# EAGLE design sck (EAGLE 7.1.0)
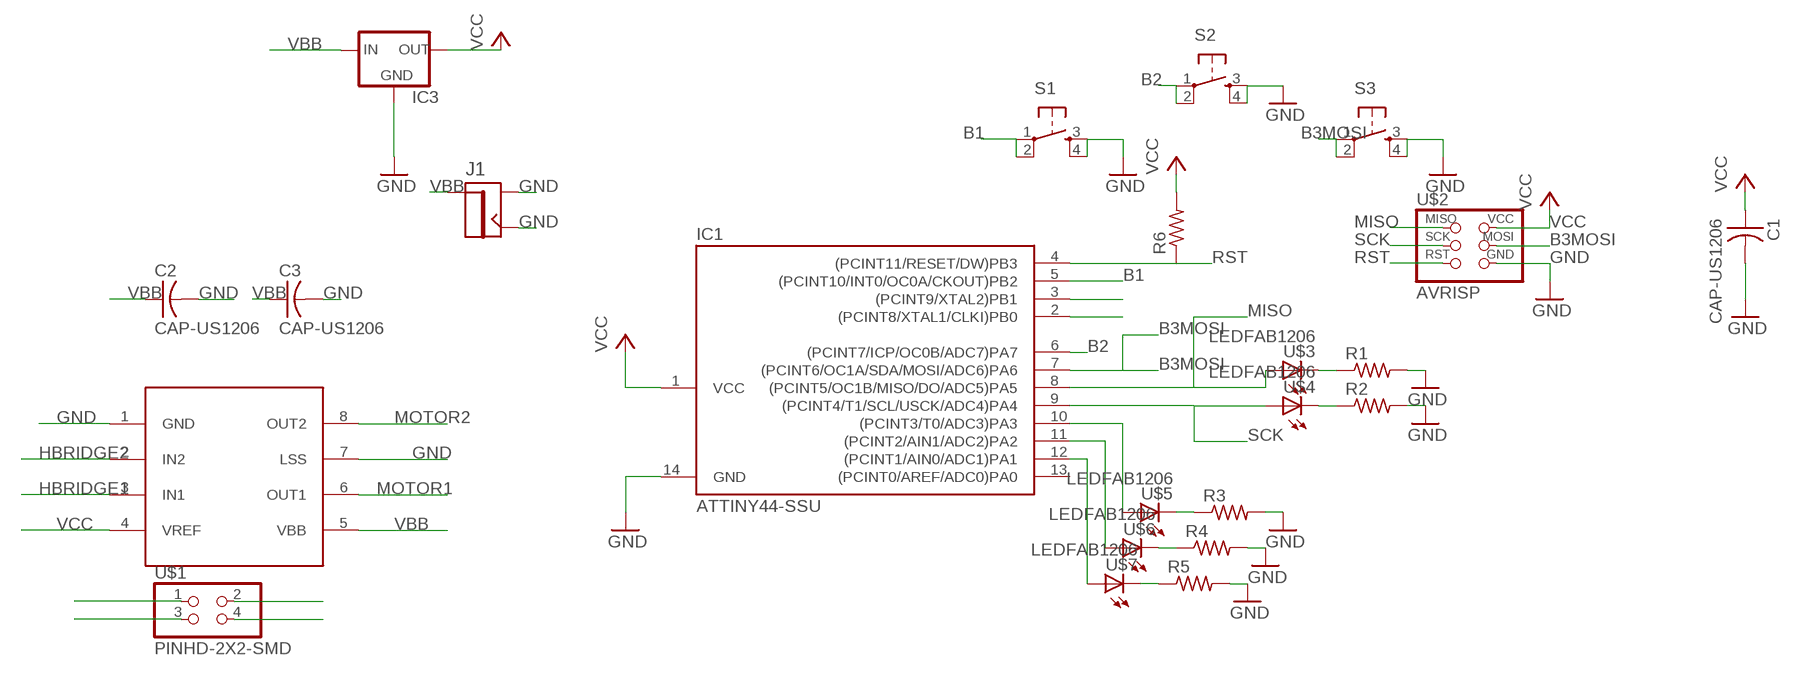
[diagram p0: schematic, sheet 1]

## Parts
C1  CAP-US1206  [C1206]
C2  CAP-US1206  [C1206]
C3  CAP-US1206  [C1206]
IC1  ATTINY44-SSU  [SOIC14]
IC3  78XXS  [78XXS]
J1  JACK2.1MM  [JACK_2.1MM]
R1  RES-US1206  [R1206]
R2  RES-US1206  [R1206]
R3  RES-US1206  [R1206]
R4  RES-US1206  [R1206]
R5  RES-US1206  [R1206]
R6  RES-US1206  [R1206]
S1  6MM_SWITCH6MM_SWITCH  [6MM_SWITCH]
S2  6MM_SWITCH6MM_SWITCH  [6MM_SWITCH]
S3  6MM_SWITCH6MM_SWITCH  [6MM_SWITCH]
U$1  PINHD-2X2-SMD  [2X02SMD]
U$2  AVRISP  [2X03]
U$3  LEDFAB1206  [LED1206FAB]
U$4  LEDFAB1206  [LED1206FAB]
U$5  LEDFAB1206  [LED1206FAB]
U$6  LEDFAB1206  [LED1206FAB]
U$7  LEDFAB1206  [LED1206FAB]
U$8  A4953-H-BRIDGE-MOTOR-DRIVER  [SOIC8]

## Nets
B1: IC1.5((PCINT10/INT0/OC0A/CKOUT)PB2) S1.1(P) S1.2(P1)
B2: IC1.6((PCINT7/ICP/OC0B/ADC7)PA7) S2.1(P) S2.2(P1)
B3MOSI: IC1.7((PCINT6/OC1A/SDA/MOSI/ADC6)PA6) S3.1(P) S3.2(P1) U$2.4(MOSI)
GND: C1.2 C2.2 C3.2 IC1.14(GND) IC3.GND J1.CONTACT J1.SHUNT R1.2 R2.2 R3.2 R4.2 R5.2 S1.3(S) S1.4(S1) S2.3(S) S2.4(S1) S3.3(S) S3.4(S1) U$2.6(GND) U$8.1(GND) U$8.7(LSS)
HBRIDGE1: IC1.2((PCINT8/XTAL1/CLKI)PB0) U$8.3(IN1)
HBRIDGE2: IC1.3((PCINT9/XTAL2)PB1) U$8.2(IN2)
MISO: IC1.8((PCINT5/OC1B/MISO/DO/ADC5)PA5) U$2.1(MISO) U$3.1(A)
MOTOR1: U$1.1 U$1.2 U$8.6(OUT1)
MOTOR2: U$1.3 U$1.4 U$8.8(OUT2)
N$1: R1.1 U$3.2(C)
N$2: R2.1 U$4.2(C)
N$3: R3.1 U$5.2(C)
N$4: R4.1 U$6.2(C)
N$5: R5.1 U$7.2(C)
N$6: IC1.12((PCINT1/AIN0/ADC1)PA1) U$7.1(A)
N$7: IC1.11((PCINT2/AIN1/ADC2)PA2) U$6.1(A)
N$8: IC1.10((PCINT3/T0/ADC3)PA3) U$5.1(A)
RST: IC1.4((PCINT11/RESET/DW)PB3) R6.1 U$2.5(RST)
SCK: IC1.9((PCINT4/T1/SCL/USCK/ADC4)PA4) U$2.3(SCK) U$4.1(A)
VBB: C2.1 C3.1 IC3.IN J1.PIN U$8.5(VBB)
VCC: C1.1 IC1.1(VCC) IC3.OUT R6.2 U$2.2(VCC) U$8.4(VREF)
Unconnected: IC1.13((PCINT0/AREF/ADC0)PA0)

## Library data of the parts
C1-C3 = fab:CAP-US
IC1 = fab:ATTINY44
IC3 = v-reg:78XXS: VOLTAGE REGULATOR
J1 = fab:JACK
R1-R6 = fab:RES-US: Resistor (US Symbol)
S1-S3 = fab:6MM_SWITCH: OMRON SWITCH
U$1 = fab:PINHD-2X2-SMD
U$2 = fab:AVRISP
U$3-U$7 = fab:LED: LED
U$8 = fab:A4953-H-BRIDGE-MOTOR-DRIVER

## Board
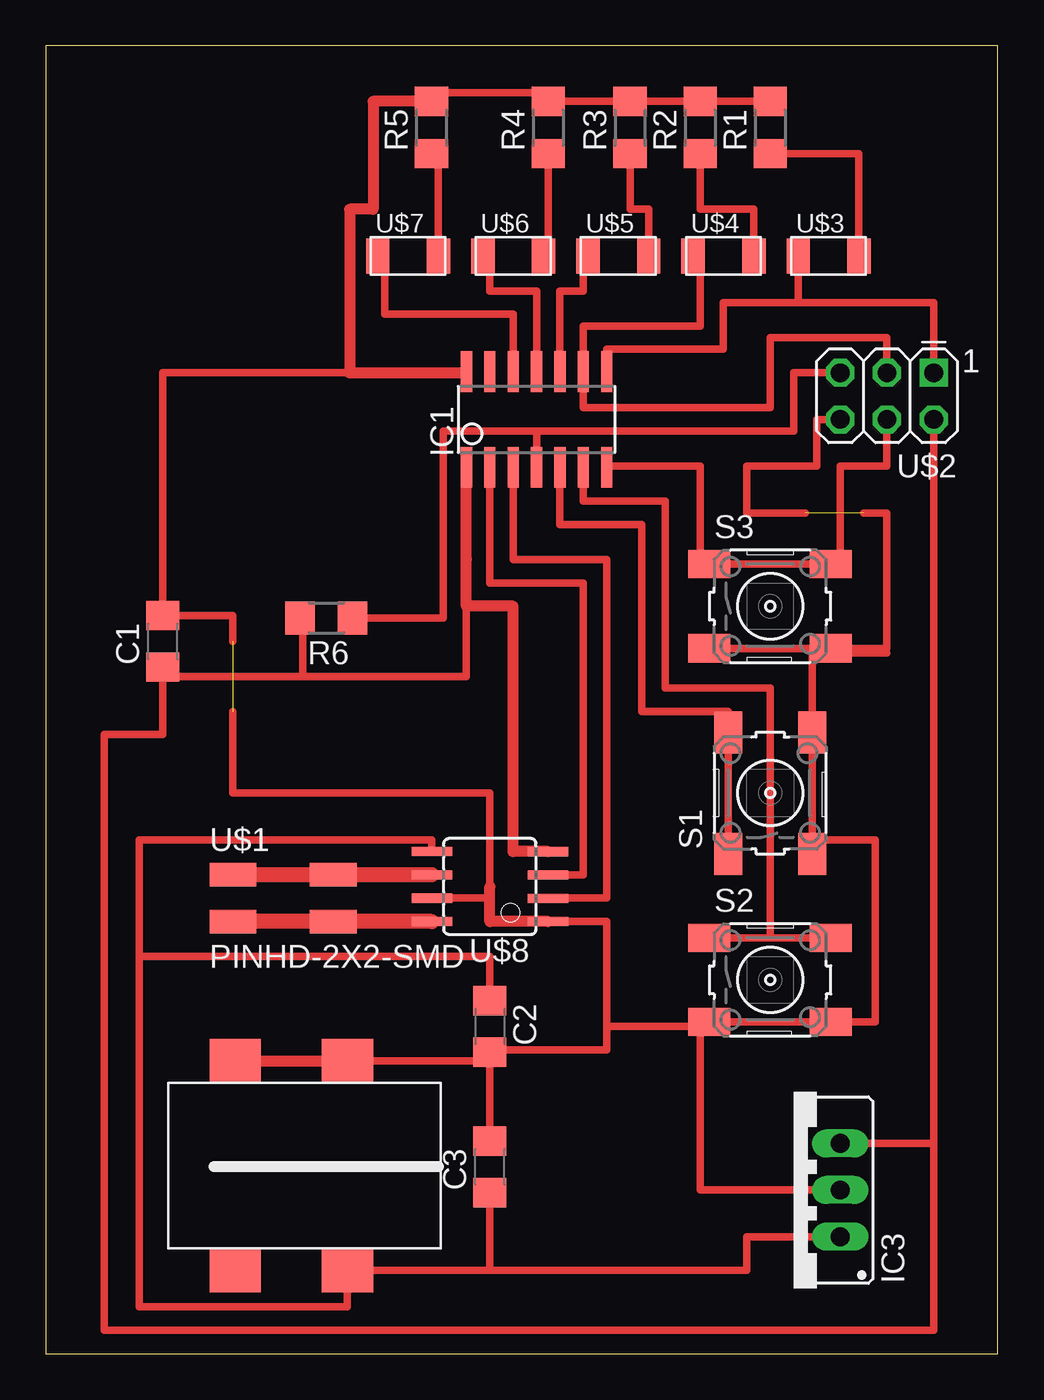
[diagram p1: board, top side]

Size 51.74 x 71.11 mm. Coordinates in mm from the lower left corner, seen from the top.
Outline: 0,0 51.74,0 51.74,71.11 0,71.11 0,0
Copper layers (1*16): Top 0.035mm / dielectric 1.5mm / Bottom 0.035mm
Design rules "default *": minimum track width 10mil, minimum drill 24mil, track to track 16mil, track to pad 16mil, pad to pad 8mil, via to via 8mil, smd to smd 8mil, copper to edge 40mil, drill to drill 8mil, minimum pad ring 10mil, minimum via ring 8mil, stop-mask expansion 4mil, vias tented up to drill 0mil, thermal gap 10mil

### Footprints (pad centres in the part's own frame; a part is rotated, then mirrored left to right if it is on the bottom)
C1206 = smd 1.6 x 1.8: 1 -1.4,0; 2 1.4,0
SOIC14 = smd 0.61 x 2.21: 1 -3.81,-2.603; 2 -2.54,-2.603; 3 -1.27,-2.603; 4 0,-2.603; 5 1.27,-2.603; 6 2.54,-2.603; 7 3.81,-2.603; 8 3.81,2.603; 9 2.54,2.603; 10 1.27,2.603; 11 0,2.603; 12 -1.27,2.603; 13 -2.54,2.603; 14 -3.81,2.603
78XXS = drill 1.016 long: GND 0,-2.54; IN -2.54,-2.54; OUT 2.54,-2.54
JACK_2.1MM = smd 2.388 x 2.794: CONTACT 5.766,-2.413; PIN -5.639,-2.413; PIN1 -5.639,3.683; SHUNT 5.766,3.683
R1206 = smd 1.6 x 1.803: 1 -1.422,0; 2 1.422,0
6MM_SWITCH = smd 2.286 x 1.524: 1 -3.302,2.286; 2 3.302,2.286; 3 -3.302,-2.286; 4 3.302,-2.286
2X02SMD = smd 2.54 x 1.27: 1 -2.54,1.27; 2 2.92,1.27; 3 -2.54,-1.27; 4 2.92,-1.27
2X03 = drill 1.016 square: 1 -2.54,-1.27 | drill 1.016 octagon: 2 -2.54,1.27; 3 0,-1.27; 4 0,1.27; 5 2.54,-1.27; 6 2.54,1.27
LED1206FAB = smd 1.27 x 1.905: 1 -1.651,0; 2 1.651,0
SOIC8 = smd 0.5 x 2.2: 1 -1.905,-3.154; 2 -0.645,-3.154; 3 0.625,-3.154; 4 1.895,-3.154; 5 1.905,3.154; 6 0.635,3.154; 7 -0.635,3.154; 8 -1.905,3.154

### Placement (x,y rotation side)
C1  6.35,38.73 90 top
C2  24.13,17.78 270 top
C3  24.13,10.16 90 top
IC1  26.67,50.8 0 top
IC3  40.64,8.89 90 top
J1  13.97,10.16 90 top
R1  39.37,66.67 90 top
R2  35.56,66.67 90 top
R3  31.75,66.67 90 top
R4  27.3,66.67 90 top
R5  20.95,66.67 90 top
R6  15.24,40.01 180 top
S1  39.37,30.48 90 top
S2  39.37,20.32 0 top
S3  39.37,40.64 0 top
U$1  12.7,24.77 0 top
U$2  45.72,52.07 180 top
U$3  42.55,59.69 0 top
U$4  36.83,59.69 0 top
U$5  31.11,59.69 0 top
U$6  25.4,59.69 0 top
U$7  19.68,59.69 0 top
U$8  24.13,25.4 90 top

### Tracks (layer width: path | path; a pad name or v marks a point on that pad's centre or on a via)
B1
  Top 0.406: IC1.5 27.94,45.09 32.38,45.09 32.38,34.92 37.08,34.92 S1.2 S1.1
B2
  Top 0.406: S2.2 S2.1 39.37,22.61 39.37,36.2 33.66,36.2 33.66,46.35 29.21,46.35 IC1.6
B3MOSI
  Top 0.406: IC1.7 30.48,48.26 35.56,48.26 35.56,42.93 S3.1 S3.2 43.18,42.93 43.18,48.26 45.72,48.26 U$2.4
GND  (2 unrouted)
  Top 0.406: R5.2 20.95,68.58 27.3,68.58 R4.2 R3.2 R2.2 R1.2 | S3.3 S3.4 | S3.4 41.66,38.35 S1.4 41.66,27.94 | 41.66,27.94 S1.3 | U$8.1 30.48,23.5 30.48,17.78 | 30.48,17.78 35.56,17.78 | 35.56,17.78 36.07,17.78 S2.3 S2.4 45.09,18.03 45.09,27.94 41.66,27.94 | IC3.GND 35.56,8.89 35.56,17.78 | U$8.7 24.13,24.77 24.13,25.4 24.13,30.48 10.16,30.48 10.16,34.92 | C3.2 C2.2 | J1.CONTACT 24.13,15.93 C2.2 | 30.48,17.78 30.48,16.51 24.13,16.51 C2.2 | 16.51,53.34 6.35,53.34 C1.2 10.16,40.13 10.16,38.73 | 45.72,38.1 42.67,38.1 | 41.91,38.1 42.67,38.1 | 42.67,38.1 S3.4 | S3.4 45.72,38.35 45.72,45.72 44.45,45.72 | U$2.6 41.91,50.8 41.91,48.26 38.1,48.26 38.1,45.72 41.27,45.72
  Top 0.6: R5.2 17.78,68.1 17.78,62.23 16.51,62.23 16.51,53.34 22.86,53.34 IC1.14
  Top 0.61: J1.SHUNT J1.CONTACT | U$8.1 24.13,23.5 24.13,25.4
HBRIDGE1
  Top 0.406: IC1.2 24.13,41.91 29.21,41.91 29.21,26.04 27.28,26.04 U$8.3
HBRIDGE2
  Top 0.406: IC1.3 25.4,43.18 30.48,43.18 30.48,24.77 27.28,24.77 U$8.2
MISO
  Top 0.406: 40.89,57.15 U$3.1 | IC1.8 30.48,54.61 36.83,54.61 36.83,57.15 40.89,57.15 | 40.89,57.15 48.26,57.15 U$2.1
MOTOR1
  Top 0.813: U$8.6 U$1.2 U$1.1
MOTOR2
  Top 0.813: U$8.8 U$1.4 U$1.3
N$1
  Top 0.406: R1.1 44.2,65.25 U$3.2
N$2
  Top 0.406: R2.1 35.56,62.23 38.48,62.23 U$4.2
N$3
  Top 0.406: R3.1 31.75,62.23 32.77,62.23 U$5.2
N$4
  Top 0.406: U$6.2 27.3,59.69 R4.1
N$5
  Top 0.406: R5.1 21.34,65.25 U$7.2
N$6
  Top 0.406: U$7.1 18.41,59.69 18.41,56.52 25.4,56.52 IC1.12
N$7
  Top 0.406: U$6.1 24.13,59.69 24.13,57.78 26.67,57.78 IC1.11
N$8
  Top 0.406: U$5.1 29.21,59.69 29.21,57.78 27.94,57.78 IC1.10
RST
  Top 0.406: 16.51,40.01 R6.1 21.59,40.01 21.59,50.16 26.67,50.16 | 26.67,50.16 40.64,50.16 40.64,53.34 U$2.5 | IC1.4 26.67,50.16
SCK
  Top 0.406: U$4.1 35.56,59.69 35.56,55.88 29.21,55.88 IC1.9 29.21,51.44 39.37,51.44 39.37,55.24 45.72,55.24 U$2.3
VBB
  Top 0.406: 5.08,21.59 24.13,21.59 C2.1 | 5.08,21.59 5.08,2.54 16.38,2.54 J1.PIN 24.13,4.52 | 5.08,21.59 5.08,27.94 20.98,27.94 U$8.5 | 24.13,4.52 38.1,4.52 38.1,6.35 IC3.IN | C3.1 24.13,4.52
VCC
  Top 0.406: 22.86,42.55 22.86,43.18 | 22.86,40.64 22.86,36.83 13.97,36.83 | 13.97,36.83 13.97,39.37 13.82,39.37 R6.2 13.82,40.13 | U$2.2 48.26,11.43 | 6.35,36.83 6.35,33.66 3.17,33.66 3.17,1.27 48.26,1.27 48.26,11.43 | 6.35,36.83 C1.1 | 13.97,36.83 6.35,36.83 | IC3.OUT 48.26,11.43
  Top 0.6: 25.4,40.64 22.86,40.64 22.86,43.18 IC1.1
  Top 0.61: U$8.4 25.4,27.3 25.4,40.64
